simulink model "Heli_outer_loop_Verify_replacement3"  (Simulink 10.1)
settings: Solver=FixedStepDiscrete  StartTime=0.0  StopTime=10.0  RelTol=1e-3
undefined symbols (not defined in the file or in its folder): DiscIntNeverNeededParam, sldvsubsys, Ts
libraries: sldvlib x3, simulink x2

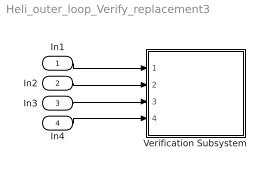
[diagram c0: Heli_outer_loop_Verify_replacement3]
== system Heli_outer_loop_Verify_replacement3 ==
  In1 : Inport
  In2 : Inport  Port=2
  In3 : Inport  Port=3
  In4 : Inport  Port=4
  Verification Subsystem : Subsystem  Tag=VerificationSubsystem  DisableCoverage=on  LoadFcn=sldvsubsys('check')  TreatAsAtomicUnit=on  SimViewingDevice=on
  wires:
  In1/1 -> Verification Subsystem/1(In1)
  In2/1 -> Verification Subsystem/2(In2)
  In3/1 -> Verification Subsystem/3(In3)
  In4/1 -> Verification Subsystem/4(In4)

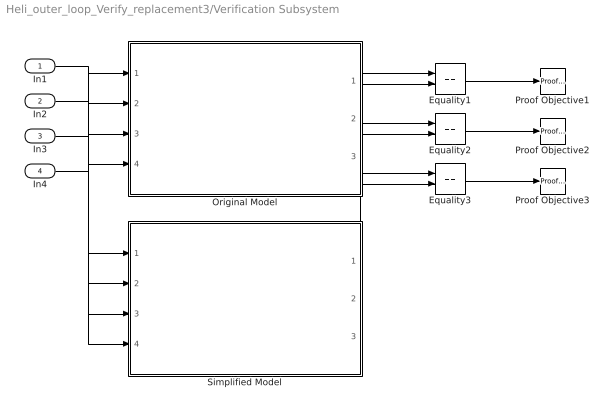
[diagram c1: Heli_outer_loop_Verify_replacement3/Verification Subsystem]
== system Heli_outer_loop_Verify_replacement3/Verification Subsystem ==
  In1 : Inport
  In2 : Inport  Port=2
  In3 : Inport  Port=3
  In4 : Inport  Port=4
  Equality1 : RelationalOperator  Operator===  OutDataTypeStr=boolean  RndMeth=Simplest
  Equality2 : RelationalOperator  Operator===  OutDataTypeStr=boolean  RndMeth=Simplest
  Equality3 : RelationalOperator  Operator===  OutDataTypeStr=boolean  RndMeth=Simplest
  Original Model : Subsystem  TreatAsAtomicUnit=on
  Proof Objective1 : sldvlib/Objectives and Constraints/Proof Objective  enabled=on  customAVTBlockType=Proof Objective  intervals=true  dispValues=on  outEnabled=off  enableStopSim=off
  Proof Objective2 : sldvlib/Objectives and Constraints/Proof Objective  enabled=on  customAVTBlockType=Proof Objective  intervals=true  dispValues=on  outEnabled=off  enableStopSim=off
  Proof Objective3 : sldvlib/Objectives and Constraints/Proof Objective  enabled=on  customAVTBlockType=Proof Objective  intervals=true  dispValues=on  outEnabled=off  enableStopSim=off
  Simplified Model : Subsystem  TreatAsAtomicUnit=on
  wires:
  In1/1 -> Original Model/1(Pilot_theta_cmd), Simplified Model/1(Pilot_theta_cmd)
  In2/1 -> Original Model/2(Pilot_phi_cmd), Simplified Model/2(Pilot_phi_cmd)
  In3/1 -> Original Model/3(Pilot_r_cmd), Simplified Model/3(Pilot_r_cmd)
  In4/1 -> Original Model/4(voted_fb), Simplified Model/4(voted_fb)
  Original Model/1(theta_cmd) -> Equality1/1
  Simplified Model/1(theta_cmd) -> Equality1/2
  Equality1/1 -> Proof Objective1/1
  Original Model/2(phi_cmd) -> Equality2/1
  Simplified Model/2(phi_cmd) -> Equality2/2
  Equality2/1 -> Proof Objective2/1
  Original Model/3(r_cmd) -> Equality3/1
  Simplified Model/3(r_cmd) -> Equality3/2
  Equality3/1 -> Proof Objective3/1

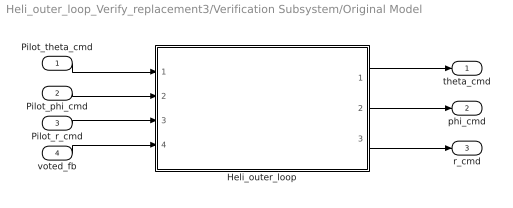
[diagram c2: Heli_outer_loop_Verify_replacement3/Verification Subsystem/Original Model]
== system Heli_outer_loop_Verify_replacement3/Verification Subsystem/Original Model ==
  Pilot_theta_cmd : Inport  OutDataTypeStr=int16  PortDimensions=1  SampleTime=[0.01,0]
  Pilot_phi_cmd : Inport  Port=2  OutDataTypeStr=int16  PortDimensions=1  SampleTime=[0.01,0]
  Pilot_r_cmd : Inport  Port=3  OutDataTypeStr=int16  PortDimensions=1  SampleTime=[0.01,0]
  voted_fb : Inport  Port=4  OutDataTypeStr=double  PortDimensions=5  SampleTime=[0.01,0]
  Heli_outer_loop : Subsystem  TreatAsAtomicUnit=on
  theta_cmd : Outport  OutDataTypeStr=double  PortDimensions=1  SampleTime=[0.01,0]
  phi_cmd : Outport  Port=2  OutDataTypeStr=double  PortDimensions=1  SampleTime=[0.01,0]
  r_cmd : Outport  Port=3  OutDataTypeStr=double  PortDimensions=1  SampleTime=[0.01,0]
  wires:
  voted_fb/1 -> Heli_outer_loop/4(voted_fb)
  Heli_outer_loop/1(theta_cmd) -> theta_cmd/1
  Pilot_phi_cmd/1 -> Heli_outer_loop/2(Pilot_phi_cmd)
  Heli_outer_loop/3(r_cmd) -> r_cmd/1
  Pilot_theta_cmd/1 -> Heli_outer_loop/1(Pilot_theta_cmd)
  Pilot_r_cmd/1 -> Heli_outer_loop/3(Pilot_r_cmd)
  Heli_outer_loop/2(phi_cmd) -> phi_cmd/1

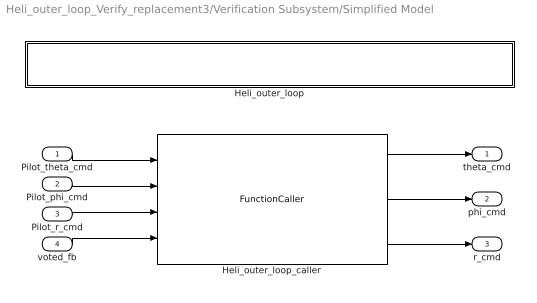
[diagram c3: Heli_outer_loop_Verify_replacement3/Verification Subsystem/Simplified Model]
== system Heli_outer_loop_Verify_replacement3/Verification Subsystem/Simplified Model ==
  Pilot_theta_cmd : Inport  OutDataTypeStr=int16  PortDimensions=1  SampleTime=[0.01,0]
  Pilot_phi_cmd : Inport  Port=2  OutDataTypeStr=int16  PortDimensions=1  SampleTime=[0.01,0]
  Pilot_r_cmd : Inport  Port=3  OutDataTypeStr=int16  PortDimensions=1  SampleTime=[0.01,0]
  voted_fb : Inport  Port=4  OutDataTypeStr=double  PortDimensions=5  SampleTime=[0.01,0]
  Heli_outer_loop : Subsystem  TreatAsAtomicUnit=on
  Heli_outer_loop_caller : FunctionCaller  FunctionPrototype=[theta_cmd,phi_cmd,r_cmd] = Heli_outer_loop(Pilot_theta_cmd,Pilot_phi_cmd,Pilot_r_cmd,voted_fb)
  theta_cmd : Outport  OutDataTypeStr=double  PortDimensions=1  SampleTime=[0.01,0]
  phi_cmd : Outport  Port=2  OutDataTypeStr=double  PortDimensions=1  SampleTime=[0.01,0]
  r_cmd : Outport  Port=3  OutDataTypeStr=double  PortDimensions=1  SampleTime=[0.01,0]
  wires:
  Heli_outer_loop_caller/3 -> r_cmd/1
  Heli_outer_loop_caller/2 -> phi_cmd/1
  Heli_outer_loop_caller/1 -> theta_cmd/1
  voted_fb/1 -> Heli_outer_loop_caller/4
  Pilot_r_cmd/1 -> Heli_outer_loop_caller/3
  Pilot_phi_cmd/1 -> Heli_outer_loop_caller/2
  Pilot_theta_cmd/1 -> Heli_outer_loop_caller/1

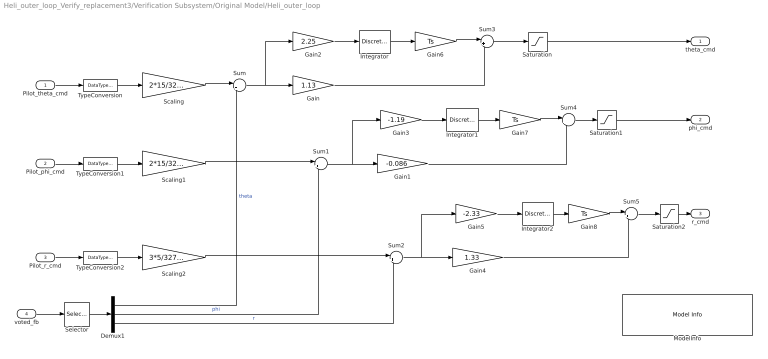
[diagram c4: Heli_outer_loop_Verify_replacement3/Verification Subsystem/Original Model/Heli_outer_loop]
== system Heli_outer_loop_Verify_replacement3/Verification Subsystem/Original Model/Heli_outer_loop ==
  Pilot_theta_cmd : Inport  OutMin=-32768  OutMax=32767  OutDataTypeStr=int16  PortDimensions=1  SampleTime=[0.01,0]
  Pilot_phi_cmd : Inport  Port=2  OutMin=-32768  OutMax=32767  OutDataTypeStr=int16  PortDimensions=1  SampleTime=[0.01,0]
  Pilot_r_cmd : Inport  Port=3  OutMin=-32768  OutMax=32767  OutDataTypeStr=int16  PortDimensions=1  SampleTime=[0.01,0]
  voted_fb : Inport  Port=4  OutMin=-180  OutMax=180  OutDataTypeStr=double  PortDimensions=5  SampleTime=[0.01,0]
  Demux1 : Demux  Outputs=3
  Gain : Gain  Gain=1.13
  Gain1 : Gain  Gain=-0.086
  Gain2 : Gain  Gain=2.25
  Gain3 : Gain  Gain=-1.19
  Gain4 : Gain  Gain=1.33
  Gain5 : Gain  Gain=-2.33
  Gain6 : Gain  Gain=Ts
  Gain7 : Gain  Gain=Ts
  Gain8 : Gain  Gain=Ts
  Integrator : DiscreteIntegrator  IntegratorMethod=Accumulation: Forward Euler  SampleTime=-1  LimitOutput=on  UpperSaturationLimit=10  LowerSaturationLimit=-10  ICPrevOutput=DiscIntNeverNeededParam  ICPrevScaledInput=DiscIntNeverNeededParam
  Integrator1 : DiscreteIntegrator  IntegratorMethod=Accumulation: Forward Euler  SampleTime=-1  LimitOutput=on  UpperSaturationLimit=10  LowerSaturationLimit=-10  ICPrevOutput=DiscIntNeverNeededParam  ICPrevScaledInput=DiscIntNeverNeededParam
  Integrator2 : DiscreteIntegrator  IntegratorMethod=Accumulation: Forward Euler  SampleTime=-1  LimitOutput=on  UpperSaturationLimit=10  LowerSaturationLimit=-10  ICPrevOutput=DiscIntNeverNeededParam  ICPrevScaledInput=DiscIntNeverNeededParam
  ModelInfo : simulink/Model-Wide Utilities/Model Info  Frame=on  DisplayStringWithTags=|  HorizontalTextAlignment=Center  LeftAlignmentValue=0.5
      | Model Name: %<ModelName>
      | Model Version: %<ModelVersion>
      | Last Modified: %<LastModificationDate>
      | 
      | Copyright 2016 The MathWorks, Inc.
  Saturation : Saturate  UpperLimit=30  LowerLimit=-30
  Saturation1 : Saturate  UpperLimit=30  LowerLimit=-30
  Saturation2 : Saturate  UpperLimit=30  LowerLimit=-30
  Scaling : Gain  Gain=2*15/32767
  Scaling1 : Gain  Gain=2*15/32767
  Scaling2 : Gain  Gain=3*5/32767
  Selector : Selector  InputPortWidth=5  IndexOptions=Index vector (dialog)  Indices=[1 2 3]  OutputSizes=1
  Sum : Sum  Inputs=|+-  InputSameDT=on
  Sum1 : Sum  Inputs=|+-  InputSameDT=on
  Sum2 : Sum  Inputs=|+-  InputSameDT=on
  Sum3 : Sum  Inputs=|++
  Sum4 : Sum  Inputs=|++
  Sum5 : Sum  Inputs=|++
  TypeConversion : DataTypeConversion  OutDataTypeStr=double
  TypeConversion1 : DataTypeConversion  OutDataTypeStr=double
  TypeConversion2 : DataTypeConversion  OutDataTypeStr=double
  theta_cmd : Outport  OutDataTypeStr=double  PortDimensions=1  SampleTime=[0.01,0]  VectorParamsAs1DForOutWhenUnconnected=off
  phi_cmd : Outport  Port=2  OutDataTypeStr=double  PortDimensions=1  SampleTime=[0.01,0]  VectorParamsAs1DForOutWhenUnconnected=off
  r_cmd : Outport  Port=3  OutDataTypeStr=double  PortDimensions=1  SampleTime=[0.01,0]  VectorParamsAs1DForOutWhenUnconnected=off
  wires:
  Gain8/1 -> Sum5/1
  Gain7/1 -> Sum4/1
  Gain6/1 -> Sum3/1
  Scaling2/1 -> Sum2/1
  Pilot_r_cmd/1 -> TypeConversion2/1
  Scaling1/1 -> Sum1/1
  Pilot_phi_cmd/1 -> TypeConversion1/1
  Scaling/1 -> Sum/1
  Pilot_theta_cmd/1 -> TypeConversion/1
  TypeConversion/1 -> Scaling/1
  TypeConversion1/1 -> Scaling1/1
  TypeConversion2/1 -> Scaling2/1
  Saturation2/1 -> r_cmd/1
  Sum2/1 -> Gain5/1, Gain4/1
  Gain5/1 -> Integrator2/1
  Integrator2/1 -> Gain8/1
  Sum5/1 -> Saturation2/1
  Gain4/1 -> Sum5/2
  Saturation1/1 -> phi_cmd/1
  Gain3/1 -> Integrator1/1
  Integrator1/1 -> Gain7/1
  Sum4/1 -> Saturation1/1
  Gain1/1 -> Sum4/2
  Sum1/1 -> Gain3/1, Gain1/1
  Saturation/1 -> theta_cmd/1
  Gain2/1 -> Integrator/1
  Integrator/1 -> Gain6/1
  Sum3/1 -> Saturation/1
  Gain/1 -> Sum3/2
  Sum/1 -> Gain/1, Gain2/1
  voted_fb/1 -> Selector/1
  Demux1/3 -> Sum2/2  "r"
  Demux1/2 -> Sum1/2  "phi"
  Demux1/1 -> Sum/2  "theta"
  Selector/1 -> Demux1/1

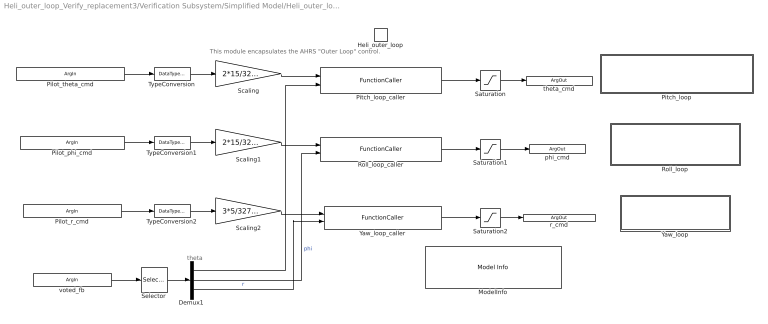
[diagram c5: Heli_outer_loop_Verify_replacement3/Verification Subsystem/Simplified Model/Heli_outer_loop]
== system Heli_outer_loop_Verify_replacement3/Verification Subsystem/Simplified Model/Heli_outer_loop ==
  note: theta
  note: This module encapsulates the AHRS "Outer Loop" control.
  Heli_outer_loop : TriggerPort  TriggerType=function-call  IsSimulinkFunction=on  FunctionName=Heli_outer_loop  FunctionVisibility=scoped  VariantControl=Variant  PortDimensions=1
  Demux1 : Demux  Outputs=3
  ModelInfo : simulink/Model-Wide Utilities/Model Info  Frame=on  DisplayStringWithTags=|  HorizontalTextAlignment=Center  LeftAlignmentValue=0.5
      | Model Name: %<ModelName>
      | Model Version: %<ModelVersion>
      | Last Modified: %<LastModificationDate>
      | 
      | Copyright 2016 The MathWorks, Inc.
  Pitch_loop : Subsystem  TreatAsAtomicUnit=on
  Pitch_loop_caller : FunctionCaller  FunctionPrototype=theta_cmd = Pitch_loop(Pilot_theta_cmd,theta)  InputArgumentSpecifications=double(1),double(1)  OutputArgumentSpecifications=double(1)
  Roll_loop : Subsystem  TreatAsAtomicUnit=on
  Roll_loop_caller : FunctionCaller  FunctionPrototype=phi_cmd = Roll_loop(Pilot_phi_cmd,phi)  InputArgumentSpecifications=double(1),double(1)  OutputArgumentSpecifications=double(1)
  Saturation : Saturate  UpperLimit=30  LowerLimit=-30
  Saturation1 : Saturate  UpperLimit=30  LowerLimit=-30
  Saturation2 : Saturate  UpperLimit=30  LowerLimit=-30
  Scaling : Gain  Gain=2*15/32767
  Scaling1 : Gain  Gain=2*15/32767
  Scaling2 : Gain  Gain=3*5/32767
  Selector : Selector  InputPortWidth=5  IndexOptions=Index vector (dialog)  Indices=[1 2 3]  OutputSizes=1
  TypeConversion : DataTypeConversion  OutDataTypeStr=double
  TypeConversion1 : DataTypeConversion  OutDataTypeStr=double
  TypeConversion2 : DataTypeConversion  OutDataTypeStr=double
  Yaw_loop : Subsystem  TreatAsAtomicUnit=on
  Yaw_loop_caller : FunctionCaller  FunctionPrototype=r_cmd = Yaw_loop(Pilot_r_cmd,r)  InputArgumentSpecifications=double(1), double(1)  OutputArgumentSpecifications=double(1)
  Pilot_theta_cmd : ArgIn  OutDataTypeStr=int16  ArgumentName=Pilot_theta_cmd
  Pilot_phi_cmd : ArgIn  Port=2  OutDataTypeStr=int16  ArgumentName=Pilot_phi_cmd
  Pilot_r_cmd : ArgIn  Port=3  OutDataTypeStr=int16  ArgumentName=Pilot_r_cmd
  voted_fb : ArgIn  Port=4  PortDimensions=5  ArgumentName=voted_fb
  theta_cmd : ArgOut  ArgumentName=theta_cmd
  phi_cmd : ArgOut  Port=2  ArgumentName=phi_cmd
  r_cmd : ArgOut  Port=3  ArgumentName=r_cmd
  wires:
  Selector/1 -> Demux1/1
  TypeConversion2/1 -> Scaling2/1
  Pilot_r_cmd/1 -> TypeConversion2/1
  Pilot_phi_cmd/1 -> TypeConversion1/1
  Saturation1/1 -> phi_cmd/1
  TypeConversion1/1 -> Scaling1/1
  Saturation2/1 -> r_cmd/1
  voted_fb/1 -> Selector/1
  Roll_loop_caller/1 -> Saturation1/1
  Yaw_loop_caller/1 -> Saturation2/1
  TypeConversion/1 -> Scaling/1
  Saturation/1 -> theta_cmd/1
  Pilot_theta_cmd/1 -> TypeConversion/1
  Scaling/1 -> Pitch_loop_caller/1
  Demux1/1 -> Pitch_loop_caller/2
  Scaling1/1 -> Roll_loop_caller/1
  Demux1/2 -> Roll_loop_caller/2  "phi"
  Pitch_loop_caller/1 -> Saturation/1
  Scaling2/1 -> Yaw_loop_caller/1
  Demux1/3 -> Yaw_loop_caller/2  "r"

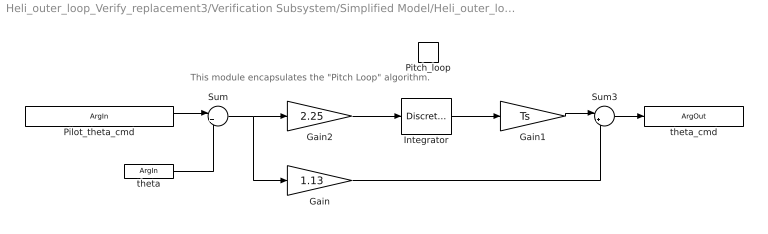
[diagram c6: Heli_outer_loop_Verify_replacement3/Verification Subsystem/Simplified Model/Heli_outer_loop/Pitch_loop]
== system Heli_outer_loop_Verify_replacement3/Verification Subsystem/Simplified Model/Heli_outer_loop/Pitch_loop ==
  note: This module encapsulates the "Pitch Loop" algorithm.
  Pitch_loop : TriggerPort  TriggerType=function-call  IsSimulinkFunction=on  FunctionName=Pitch_loop  FunctionVisibility=scoped  VariantControl=Variant  PortDimensions=1
  Gain : Gain  Gain=1.13
  Gain1 : Gain  Gain=Ts
  Gain2 : Gain  Gain=2.25
  Integrator : DiscreteIntegrator  IntegratorMethod=Accumulation: Forward Euler  SampleTime=-1  LimitOutput=on  UpperSaturationLimit=10  LowerSaturationLimit=-10  ICPrevOutput=DiscIntNeverNeededParam  ICPrevScaledInput=DiscIntNeverNeededParam
  Sum : Sum  Inputs=|+-  InputSameDT=on
  Sum3 : Sum  Inputs=|++
  Pilot_theta_cmd : ArgIn  ArgumentName=Pilot_theta_cmd
  theta : ArgIn  Port=2  ArgumentName=theta
  theta_cmd : ArgOut  ArgumentName=theta_cmd
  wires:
  Gain2/1 -> Integrator/1
  Sum3/1 -> theta_cmd/1
  Integrator/1 -> Gain1/1
  Gain/1 -> Sum3/2
  Gain1/1 -> Sum3/1
  Pilot_theta_cmd/1 -> Sum/1
  Sum/1 -> Gain/1, Gain2/1
  theta/1 -> Sum/2

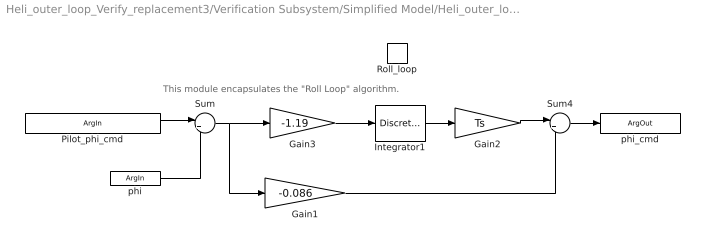
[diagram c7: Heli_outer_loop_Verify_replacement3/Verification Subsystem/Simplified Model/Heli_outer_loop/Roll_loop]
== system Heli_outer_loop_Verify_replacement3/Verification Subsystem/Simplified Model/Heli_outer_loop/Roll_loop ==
  note: This module encapsulates the "Roll Loop" algorithm.
  Roll_loop : TriggerPort  TriggerType=function-call  IsSimulinkFunction=on  FunctionName=Roll_loop  FunctionVisibility=scoped  VariantControl=Variant  PortDimensions=1
  Gain1 : Gain  Gain=-0.086
  Gain2 : Gain  Gain=Ts
  Gain3 : Gain  Gain=-1.19
  Integrator1 : DiscreteIntegrator  IntegratorMethod=Accumulation: Forward Euler  SampleTime=-1  LimitOutput=on  UpperSaturationLimit=10  LowerSaturationLimit=-10  ICPrevOutput=DiscIntNeverNeededParam  ICPrevScaledInput=DiscIntNeverNeededParam
  Sum : Sum  Inputs=|+-  InputSameDT=on
  Sum4 : Sum  Inputs=|++
  Pilot_phi_cmd : ArgIn  ArgumentName=Pilot_phi_cmd
  phi : ArgIn  Port=2  ArgumentName=phi
  phi_cmd : ArgOut  ArgumentName=phi_cmd
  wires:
  Sum4/1 -> phi_cmd/1
  Gain3/1 -> Integrator1/1
  Gain1/1 -> Sum4/2
  Integrator1/1 -> Gain2/1
  Gain2/1 -> Sum4/1
  phi/1 -> Sum/2
  Pilot_phi_cmd/1 -> Sum/1
  Sum/1 -> Gain1/1, Gain3/1

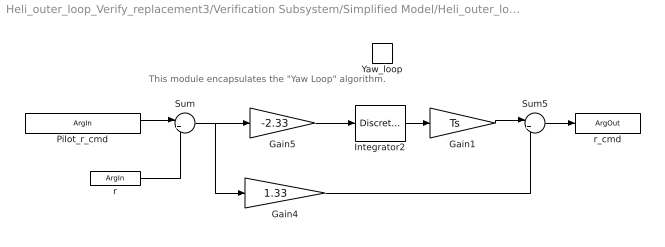
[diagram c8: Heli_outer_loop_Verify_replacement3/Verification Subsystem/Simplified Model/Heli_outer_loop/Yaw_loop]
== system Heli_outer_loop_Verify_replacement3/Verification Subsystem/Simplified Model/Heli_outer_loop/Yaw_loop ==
  note: This module encapsulates the "Yaw Loop" algorithm.
  Yaw_loop : TriggerPort  TriggerType=function-call  IsSimulinkFunction=on  FunctionName=Yaw_loop  FunctionVisibility=scoped  VariantControl=Variant  PortDimensions=1
  Gain1 : Gain  Gain=Ts
  Gain4 : Gain  Gain=1.33
  Gain5 : Gain  Gain=-2.33
  Integrator2 : DiscreteIntegrator  IntegratorMethod=Accumulation: Forward Euler  SampleTime=-1  LimitOutput=on  UpperSaturationLimit=10  LowerSaturationLimit=-10  ICPrevOutput=DiscIntNeverNeededParam  ICPrevScaledInput=DiscIntNeverNeededParam
  Sum : Sum  Inputs=|+-  InputSameDT=on
  Sum5 : Sum  Inputs=|++
  Pilot_r_cmd : ArgIn  ArgumentName=Pilot_r_cmd
  r : ArgIn  Port=2  ArgumentName=r
  r_cmd : ArgOut  ArgumentName=r_cmd
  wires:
  Integrator2/1 -> Gain1/1
  Gain4/1 -> Sum5/2
  Gain5/1 -> Integrator2/1
  Sum5/1 -> r_cmd/1
  Gain1/1 -> Sum5/1
  r/1 -> Sum/2
  Pilot_r_cmd/1 -> Sum/1
  Sum/1 -> Gain4/1, Gain5/1
